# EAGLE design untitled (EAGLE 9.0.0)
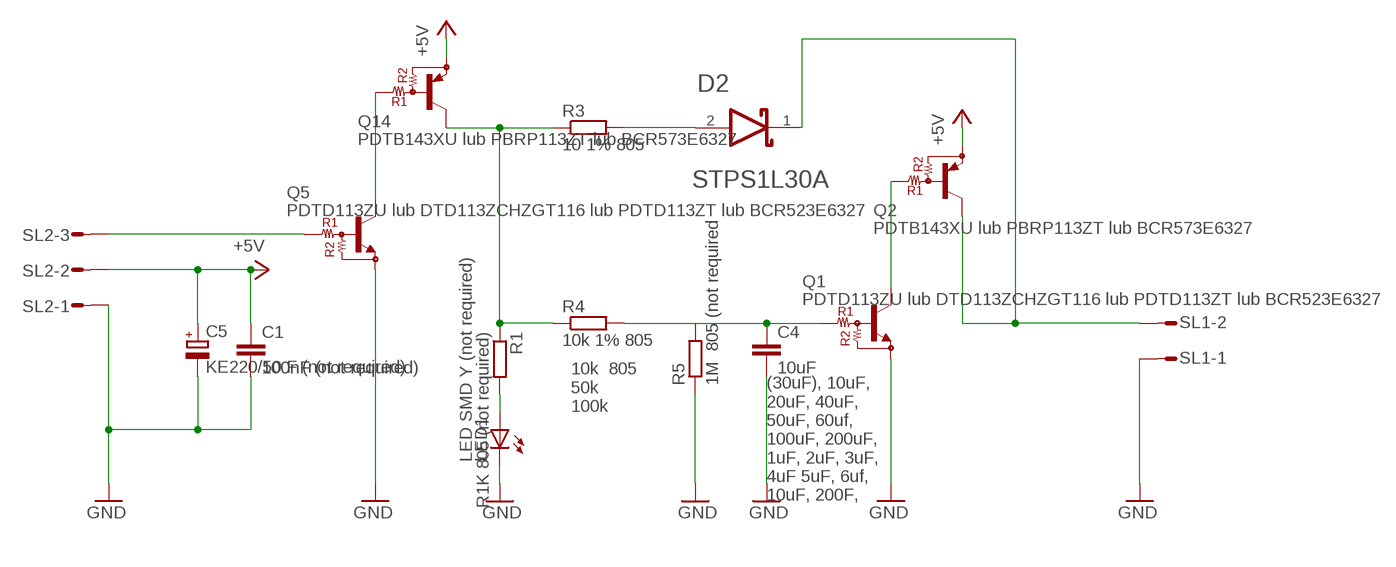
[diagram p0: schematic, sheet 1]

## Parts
C1  100nF (not required)  C-EUC0805  [C0805]
C4  10uF  C-EUC0805  [C0805]
C5  KE220/50 F (not required)  CPOL-EUG  [PANASONIC_G]
D2  MBR0530T1G, STPS1L30A lub STPS1L30U  STMICROELECTRONICS_STPS1L30ASTMICROELECTRONICS_STPS1L30A_0_0  [STMICROELECTRONICS_STPS1L30A_0]
LED1  LED SMD Y (not required)  LEDCHIP-LED0805  [CHIP-LED0805]
Q1  PDTD113ZU lub DTD113ZCHZGT116 lub PDTD113ZT lub BCR523E6327  PDTD113ZU  [SOT-23]
Q2  PDTB143XU lub PBRP113ZT lub BCR573E6327  PDTB143XU  [SOT-23]
Q5  PDTD113ZU lub DTD113ZCHZGT116 lub PDTD113ZT lub BCR523E6327  PDTD113ZU  [SOT-23]
Q14  PDTB143XU lub PBRP113ZT lub BCR573E6327  PDTB143XU  [SOT-23]
R1  R1K 805 (not required)  R-EU_R0805  [R0805]
R3  10 1% 805  R-EU_M0805  [M0805]
R4  10k 1% 805  R-EU_M0805  [M0805]
R5  1M 805 (not required  R-EU_M0805  [M0805]
SL1  M02S  [02P]
SL2  M03S  [03P]

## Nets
+5V: C1.1 C5.+ Q2.2(E) Q14.2(E) SL2.2
GND: C1.2 C4.2 C5.- LED1.C Q1.2(E) Q5.2(E) R5.1 SL1.1 SL2.1
N$1: Q1.3(C) Q2.1(B)
N$2: LED1.A R1.2
N$4: Q14.3(C) R1.1 R3.1 R4.1
N$5: D2.2(ANODE) R3.2
N$6: Q5.1(B) SL2.3
N$7: Q5.3(C) Q14.1(B)
N$8: C4.1 Q1.1(B) R4.2 R5.2
SOFT_START_5.0V: D2.1(CATHODE) Q2.3(C) SL1.2

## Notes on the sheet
- 10k  805
  50k 
  100k
- (30uF), 10uF,
  20uF, 40uF,
  50uF, 60uf,
  100uF, 200uF,
  1uF, 2uF, 3uF,
  4uF 5uF, 6uf,
  10uF, 200F,

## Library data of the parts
C1 C4 = rcl:C-EU: CAPACITOR, European symbol
C5 = rcl:CPOL-EU: POLARIZED CAPACITOR, European symbol
D2 = STMicroelectronics - STPS1L30A:STMICROELECTRONICS_STPS1L30A: LOW DROP POWER SCHOTTKY RECTIFIER; CENTROID_NOT_SPECIFIED: No; DATASHEET: http://www.st.com/content/ccc/resource/technical/document/datasheet/d4/83/f4/ff/dc/cc/48/7f/CD00001323.pdf/files/CD00001323.pdf/jcr:content/translations/en.CD00001323.pdf; DIGIKEY_DESCRIPTION: DIODE SCHOTTKY 30V 1A SMA; DIGIKEY_PART_NUMBER: 497-6577-1-ND; LEAD_FREE: yes; MF: STMicroelectronics; MOUSER_PART_NUMBER: 511-STPS1L30A; MPN: STPS1L30A; PACKAGE: DO-214AC; PREFIX: D; ROHS: yes; TEMPERATURE_RANGE_HIGH: +150°C
LED1 = adafruit:LED: LED
Q1 Q5 = pre-bias-transistor:PDTD: Pre biase NPN transistor NPN Resistor-Equipped Transistor (RET) family in a very small SOT323 (SC-70) Surface-Mounted Device (SMD) plastic package. VCC = 50V Ic (max) = 500 mA; R1: 1 kOhm; R2: 10 kOhm
Q2 Q14 = pre-bias-transistor:PDTB: PNP Resistor-Equipped Transistor (RET) family in a very small SOT323 (SC-70) Surface-Mounted Device (SMD) plastic package. VCC = -50 IC (max) = -500mA; R1: 4.7 kOhm; R2: 10 kOhm
R1 R3-R5 = rcl:R-EU_: RESISTOR, European symbol
SL1 = con-amp-quick:M02S: AMP QUICK CONNECTOR; OC_FARNELL: unknown; OC_NEWARK: unknown
SL2 = con-amp-quick:M03S: AMP QUICK CONNECTOR; OC_FARNELL: unknown; OC_NEWARK: unknown

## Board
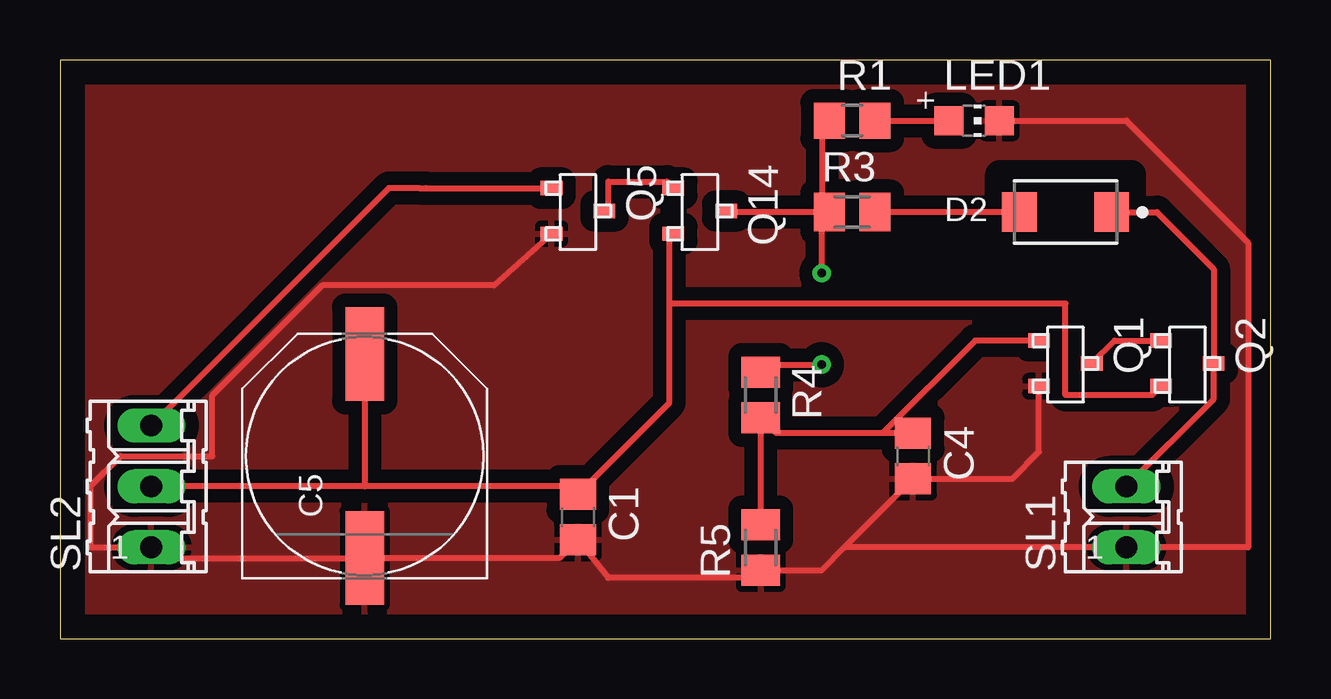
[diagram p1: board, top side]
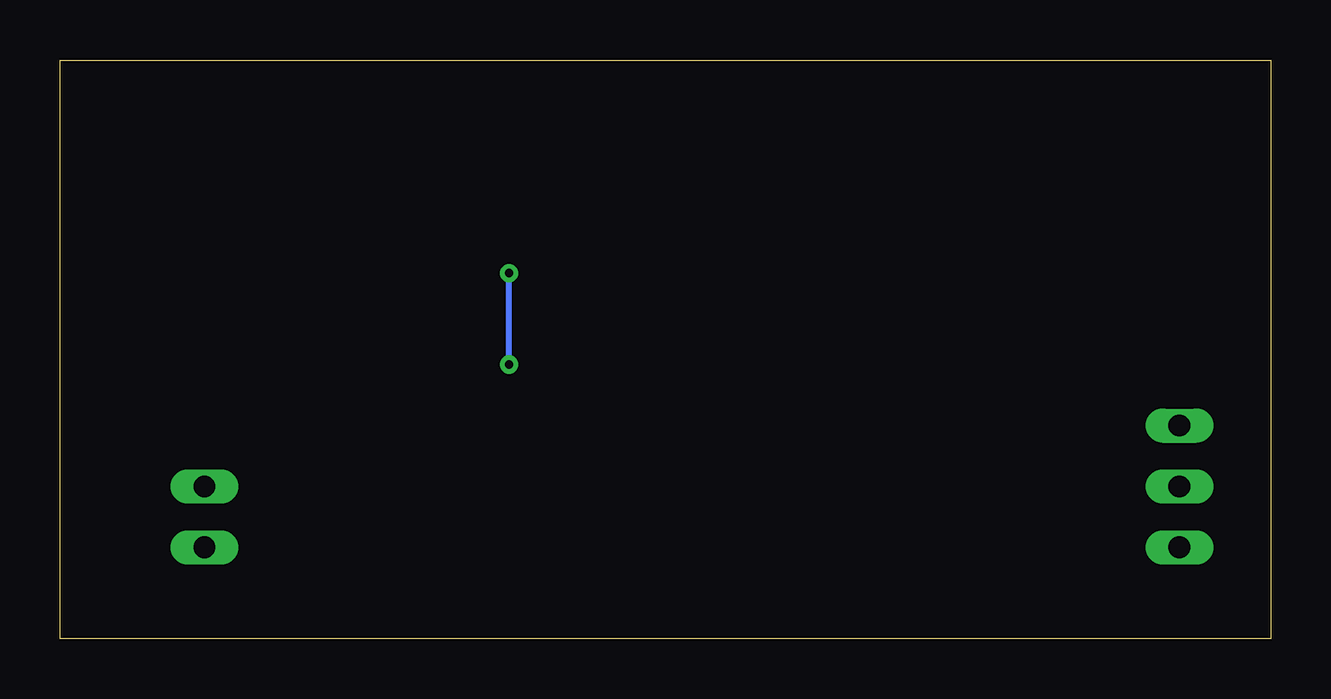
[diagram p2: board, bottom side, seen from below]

Size 50.47 x 24.12 mm. Coordinates in mm from the lower left corner, seen from the top.
Outline: 0,0 50.47,0 50.47,24.12 0,24.12 0,0
Copper layers (1*16): Top 0.035mm / dielectric 1.5mm / Bottom 0.035mm
Design rules "default": minimum track width 6mil, minimum drill 0.35mm, track to track 6mil, track to pad 6mil, pad to pad 6mil, via to via 6mil, smd to smd 6mil, copper to edge 40mil, drill to drill 6mil, minimum pad ring 10mil, minimum via ring 8mil, stop-mask expansion 4mil, vias tented up to drill 0mil, thermal gap 10mil

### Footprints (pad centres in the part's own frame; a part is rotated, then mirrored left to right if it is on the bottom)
C0805 = smd 1.3 x 1.5: 1 -0.95,0; 2 0.95,0
PANASONIC_G = smd 3.9 x 1.6: + 4.25,0; - -4.25,0
STMICROELECTRONICS_STPS1L30A_0 = smd 1.45 x 1.65: 1 -1.925,0; 2 1.925,0
CHIP-LED0805 = smd 1.2 x 1.2: A 0,-1.05; C 0,1.05
SOT-23 = smd 0.6 x 0.9: 1 -1,-1.1; 2 0.9,-1.1; 3 -0.05,1.1
R0805 = smd 1.3 x 1.5: 1 -0.95,0; 2 0.95,0
M0805 = smd 1.3 x 1.6: 1 -0.95,0; 2 0.95,0
02P = drill 0.914 long: 1 -1.27,0; 2 1.27,0
03P = drill 0.914 long: 1 -2.54,0; 2 0,0; 3 2.54,0

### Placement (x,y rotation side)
C1  21.59,5.08 270 top
C4  35.56,7.62 270 top
C5  12.7,7.62 90 top
D2  41.91,17.78 180 top
LED1  38.1,21.59 270 top
Q1  41.91,11.43 270 top
Q2  46.99,11.43 270 top
Q5  21.59,17.78 270 top
Q14  26.67,17.78 270 top
R1  33.02,21.59 0 top
R3  33.02,17.78 0 top
R4  29.21,10.16 270 top
R5  29.21,3.81 90 top
SL1  44.45,5.08 90 top
SL2  3.81,6.35 90 top

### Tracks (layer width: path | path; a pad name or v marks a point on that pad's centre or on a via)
+5V
  Top 0.254: 12.7,10.16 C5.+ 12.7,6.35 | 12.7,6.35 21.27,6.35 C1.1 25.4,9.84 25.4,13.97 | 12.7,6.35 SL2.2 | Q2.2 45.52,10.16 41.91,10.16 41.91,13.97 25.4,13.97 | 25.4,13.97 25.4,16.71 Q14.2
GND
  Top 0.254: 32.7,3.81 C4.2 39.69,6.67 40.81,7.79 Q1.2 | 32.7,3.81 SL1.1 49.53,3.81 49.53,16.51 44.45,21.59 LED1.C | 32.7,3.81 31.75,2.86 R5.1 28.89,2.54 22.86,2.54 C1.2 20.83,3.37 C5.- 4.25,3.37 SL2.1 1.27,3.81 1.27,6.35 2.54,7.62 6.35,7.62 6.35,10.16 10.92,14.73 18.09,14.73 Q5.2
  pour Top (isolate 0.559): -1.27,12.7 -1.27,25.4 52.07,25.4 52.07,-1.27 -1.27,-1.27
N$1
  Top 0.254: Q1.3 43.96,12.43 Q2.1
N$2
  Top 0.254: R1.2 LED1.A
N$4  (via drill 0.35)
  Top 0.254: R3.1 31.75,17.78 | 31.75,17.78 27.82,17.78 Q14.3 | R1.1 31.75,21.27 31.75,17.78 | R4.1 29.53,11.43 v31.75,11.43 | v31.75,15.24 31.75,17.78
  Bottom 0.254: v31.75,11.43 v31.75,15.24
N$5
  Top 0.254: D2.2 R3.2
N$6
  Top 0.254: Q5.1 15.24,18.78 14.97,18.78 13.7,18.78 SL2.3
N$7
  Top 0.254: Q5.3 22.86,18 22.86,19.05 25.3,19.05 Q14.1
N$8
  Top 0.254: C4.1 34.29,8.57 | 34.29,8.57 29.85,8.57 R4.2 R5.2 | Q1.1 38.15,12.43 34.29,8.57
SOFT_START_5.0V
  Top 0.254: SL1.2 48.09,9.99 Q2.3 48.09,15.41 45.72,17.78 D2.1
